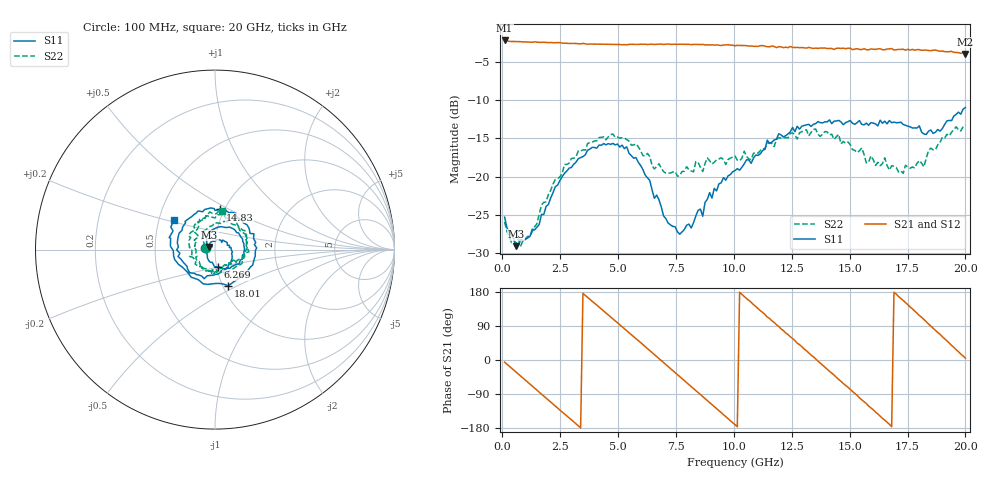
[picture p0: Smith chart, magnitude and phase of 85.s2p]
!Agilent Technologies,N5230C,MY49001569,A.09.33.09
!Agilent N5230C: A.09.33.09
!Date: Friday, July 24, 2015 10:07:38
!Correction: S11(Full 2 Port(1,2))
!S21(Full 2 Port(1,2))
!S12(Full 2 Port(1,2))
!S22(Full 2 Port(1,2))
!S2P File: Measurements: S11, S21, S12, S22:
# Hz S  dB  R 50
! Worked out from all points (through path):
!   201 points, 100 MHz to 20 GHz, reference 50 ohm
!   highest |S21| = -2.20 dB at 100 MHz (marker M1); lowest = -4.0 dB at 20 GHz (marker M2)
!   group delay of S21, straight-line fit = 149 ps
!   lowest |S11| = -29.1 dB at 597.5 MHz (marker M3), VSWR 1.07, Z = 46.9 + j1.44 ohm
!   |S11| at or under -10 dB: start of sweep to end of sweep
!   |S22| runs from -29.0 to -13.3 dB; largest |S21 - S12| = 0.02
!   S11 on the Smith chart (normalised r, x): 100 MHz: 0.90, +0.01; 6.269 GHz: 1.01, -0.20; 14.83 GHz: 0.95, +0.45; 18.01 GHz: 1.06, -0.45; 20 GHz: 0.60, +0.21
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1e8  -25.30 171.5  -2.20 -5.7  -2.18 -5.5  -25.93 170.2
5.975e8  -29.09 154.1  -2.34 -32.2  -2.35 -32.1  -28.74 161.3
1.891e9  -23.89 138.0  -2.45 -100.5  -2.46 -100.8  -23.28 151.9
2.687e9  -19.56 106.1  -2.55 -142.4  -2.52 -142.7  -18.39 121.2
3.483e9  -17.38 66.7  -2.58 175.8  -2.63 175.8  -16.49 85.8
4.876e9  -15.85 -4.7  -2.73 103.5  -2.72 103.4  -14.85 21.5
6.269e9  -20.15 -81.8  -2.73 30.2  -2.70 30.1  -16.96 -33.0
6.7665e9  -23.01 -119.1  -2.68 3.8  -2.69 3.9  -18.32 -41.0
7.662e9  -27.52 139.2  -2.69 -43.8  -2.70 -43.6  -19.87 -61.7
8.458e9  -24.40 63.7  -2.72 -86.1  -2.77 -85.9  -18.14 -83.3
9.1545e9  -21.53 16.5  -2.82 -123.0  -2.79 -123.3  -18.12 -109.0
1.005e10  -19.21 -33.7  -2.89 -170.5  -2.85 -170.9  -17.30 -144.6
1.07465e10  -18.27 -73.3  -2.92 152.2  -2.88 151.7  -17.78 178.5
1.17415e10  -15.21 -126.4  -2.98 99.0  -2.94 97.9  -16.07 136.4
1.2438e10  -14.13 -164.1  -2.98 61.3  -3.04 61.2  -14.32 105.5
1.3433e10  -13.16 145.2  -3.24 8.6  -3.21 8.3  -13.83 57.0
1.4826e10  -12.94 82.9  -3.28 -66.7  -3.28 -67.0  -15.63 -21.9
1.57215e10  -13.00 47.7  -3.40 -115.1  -3.23 -116.0  -18.21 -80.0
1.67165e10  -12.66 2.1  -3.31 -169.6  -3.43 -170.3  -19.13 -143.3
1.801e10  -13.36 -69.6  -3.40 117.4  -3.49 118.1  -17.89 155.4
1.89055e10  -14.05 -140.5  -3.59 67.8  -3.59 67.2  -15.54 122.4
2e10  -10.97 144.3  -3.95 4.8  -3.96 4.8  -13.27 80.1
